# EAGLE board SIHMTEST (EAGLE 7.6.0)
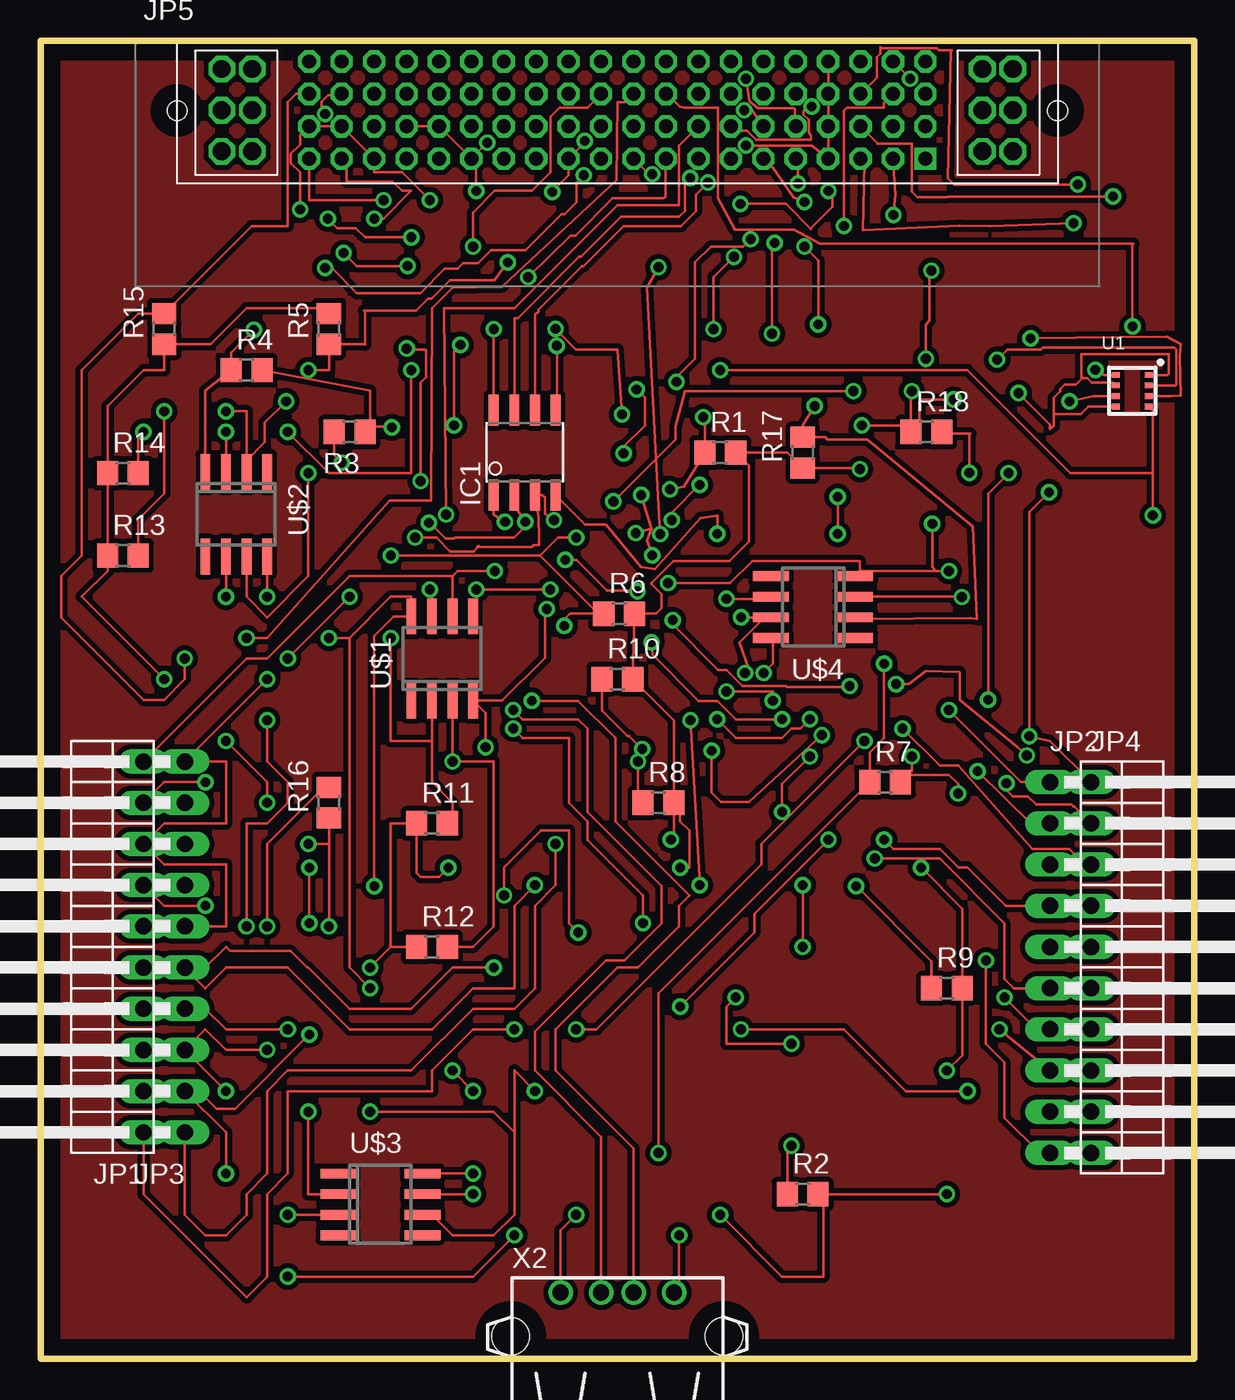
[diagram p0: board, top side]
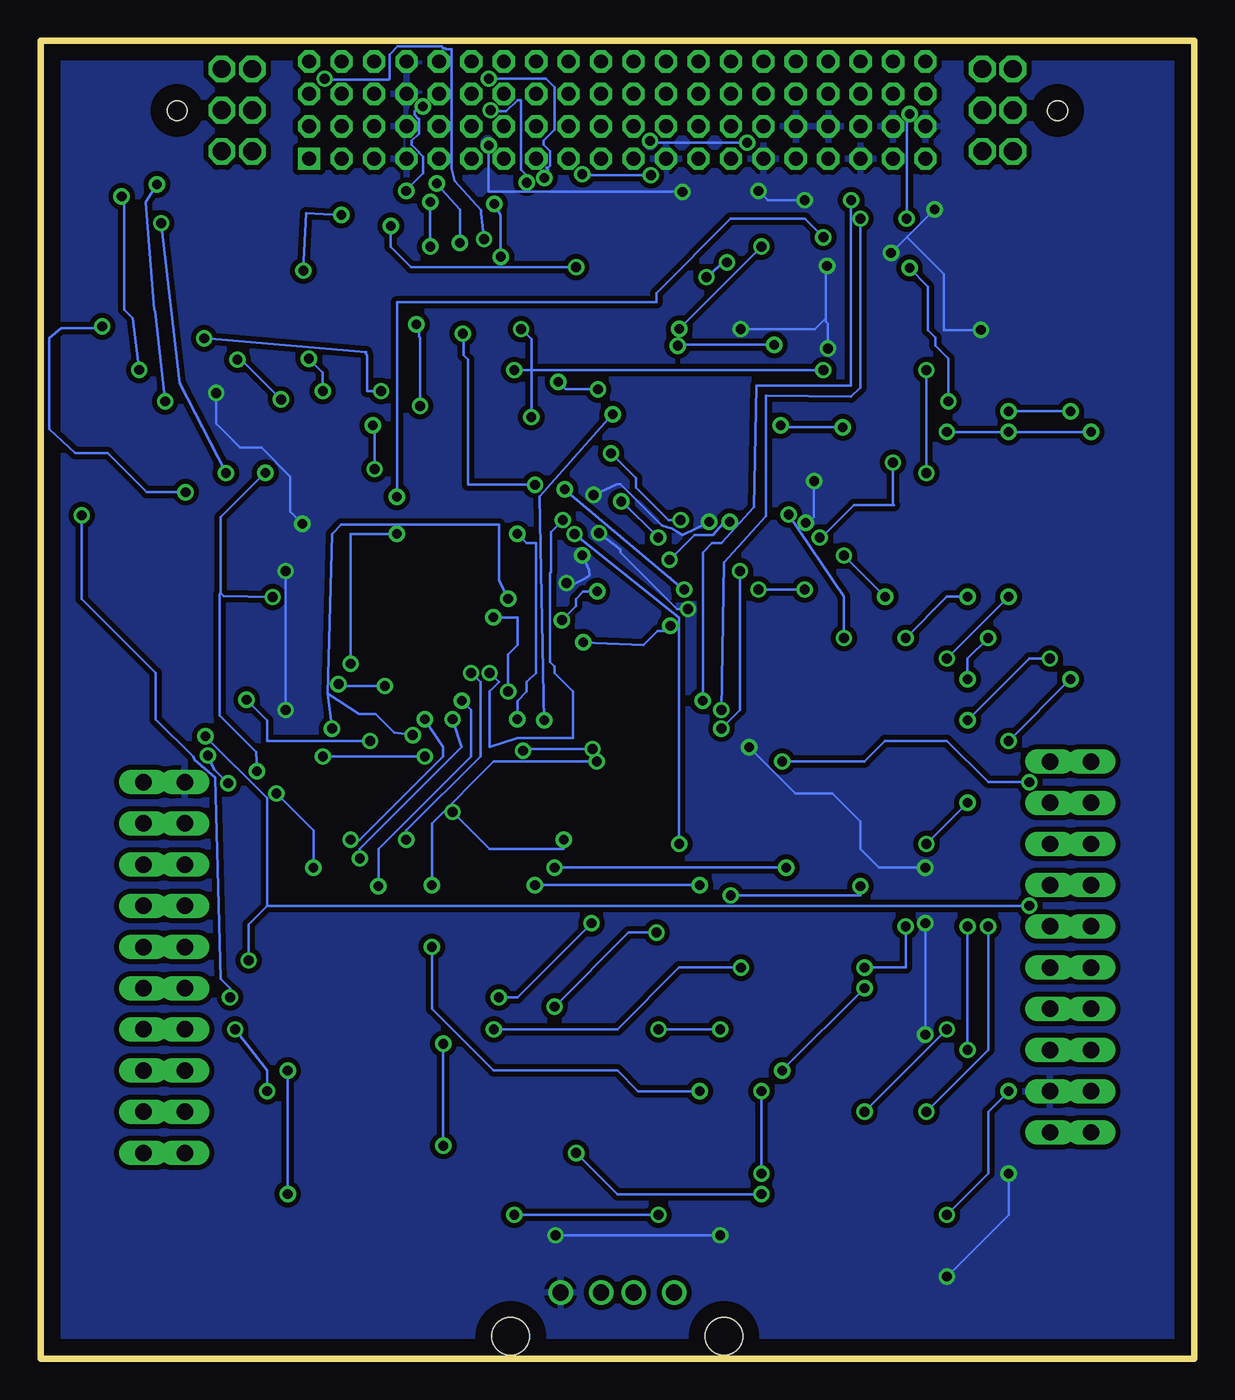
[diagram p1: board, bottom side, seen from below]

Size 71.12 x 81.28 mm. Coordinates in mm from the lower left corner, seen from the top.
Outline: 0,0 0,81.28 71.12,81.28 71.12,0 0,0
Copper layers (1*16): Top 0.035mm / dielectric 1.5mm / Bottom 0.035mm
Design rules "default": minimum track width 10mil, minimum drill 24mil, track to track 8mil, track to pad 8mil, pad to pad 8mil, via to via 8mil, smd to smd 8mil, copper to edge 40mil, drill to drill 8mil, minimum pad ring 10mil, minimum via ring 8mil, stop-mask expansion 4mil, vias tented up to drill 0mil, thermal gap 10mil

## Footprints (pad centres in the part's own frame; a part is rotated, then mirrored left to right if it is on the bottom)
SO08 = smd 0.61 x 1.905: 1 -1.905,-2.616; 2 -0.635,-2.616; 3 0.635,-2.616; 4 1.905,-2.616; 5 1.905,2.616; 6 0.635,2.616; 7 -0.635,2.616; 8 -1.905,2.616
1X10/90 = drill 1.016 long: 1 -11.43,-3.81; 2 -8.89,-3.81; 3 -6.35,-3.81; 4 -3.81,-3.81; 5 -1.27,-3.81; 6 1.27,-3.81; 7 3.81,-3.81; 8 6.35,-3.81; 9 8.89,-3.81; 10 11.43,-3.81
MPSC-01-80 = drill 0.86 square: 1 19,0.33 | drill 0.86 octagon: 2 17,0.33; 3 15,0.33; 4 13,0.33; 5 11,0.33; 6 9,0.33; 7 7,0.33; 8 5,0.33; 9 3,0.33; 10 1,0.33; 11 -1,0.33; 12 -3,0.33; 13 -5,0.33; 14 -7,0.33; 15 -9,0.33; 16 -11,0.33; 17 -13,0.33; 18 -15,0.33; 19 -17,0.33; 20 -19,0.33; 21 19,2.33; 22 17,2.33; 23 15,2.33; 24 13,2.33; 25 11,2.33; 26 9,2.33; 27 7,2.33; 28 5,2.33; 29 3,2.33; 30 1,2.33; 31 -1,2.33; 32 -3,2.33; 33 -5,2.33; 34 -7,2.33; 35 -9,2.33; 36 -11,2.33; 37 -13,2.33; 38 -15,2.33; 39 -17,2.33; 40 -19,2.33; 41 19,4.33; 42 17,4.33; 43 15,4.33; 44 13,4.33; 45 11,4.33; 46 9,4.33; 47 7,4.33; 48 5,4.33; 49 3,4.33; 50 1,4.33; 51 -1,4.33; 52 -3,4.33; 53 -5,4.33; 54 -7,4.33; 55 -9,4.33; 56 -11,4.33; 57 -13,4.33; 58 -15,4.33; 59 -17,4.33; 60 -19,4.33; 61 19,6.33; 62 17,6.33; 63 15,6.33; 64 13,6.33; 65 11,6.33; 66 9,6.33; 67 7,6.33; 68 5,6.33; 69 3,6.33; 70 1,6.33; 71 -1,6.33; 72 -3,6.33; 73 -5,6.33; 74 -7,6.33; 75 -9,6.33; 76 -11,6.33; 77 -13,6.33; 78 -15,6.33; 79 -17,6.33; 80 -19,6.33 | drill 1.1 octagon: P1,1 -24.385,0.79; P1,2 -22.505,0.79; P1,3 -24.385,3.33; P1,4 -22.505,3.33; P1,5 -24.385,5.87; P1,6 -22.505,5.87; P2,1 24.385,0.789; P2,2 22.505,0.789; P2,3 24.385,3.329; P2,4 22.505,3.329; P2,5 24.385,5.869; P2,6 22.505,5.869 | hole 1.2: -27.145,3.3; 27.145,3.3
R0805 = smd 1.3 x 1.5: 1 -0.95,0; 2 0.95,0
BME280_LGA = smd 0.5 x 0.35: P$1 1.025,0.975; P$2 1.025,0.325; P$3 1.025,-0.325; P$4 1.025,-0.975; P$5 -1.025,-0.975; P$6 -1.025,-0.325; P$7 -1.025,0.325; P$8 -1.025,0.975
SO8 = smd 0.6 x 2.2: 1 -1.905,-2.6; 2 -0.635,-2.6; 3 0.635,-2.6; 4 1.905,-2.6; 5 1.905,2.6; 6 0.635,2.6; 7 -0.635,2.6; 8 -1.905,2.6
USB = drill 1: 1 -3.5,12.99; 2 -1,12.99; 3 1,12.99; 4 3.5,12.99 | hole 2.3: -6.57,10.28; 6.57,10.28

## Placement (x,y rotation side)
IC1  MCP2551/SN  [SO08]  29.84,55.88 0 top
JP1  [1X10/90]  2.54,25.4 90 top
JP2  [1X10/90]  66.04,24.13 270 top
JP3  [1X10/90]  5.08,25.4 90 top
JP4  [1X10/90]  68.58,24.13 270 top
JP5  [MPSC-01-80]  35.56,73.66 0 top
R1  5k  [R0805]  41.91,55.88 0 top
R2  5k  [R0805]  46.99,10.16 0 top
R3  10k  [R0805]  19.05,57.15 180 top
R4  10k  [R0805]  12.7,60.96 0 top
R5  5k  [R0805]  17.78,63.5 90 top
R6  5k  [R0805]  35.67,45.95 0 top
R7  5k  [R0805]  52.07,35.56 0 top
R8  5k  [R0805]  38.1,34.29 0 top
R9  5k  [R0805]  55.88,22.86 0 top
R10  5k  [R0805]  35.56,41.91 0 top
R11  5k  [R0805]  24.13,33.02 0 top
R12  5k  [R0805]  24.13,25.4 0 top
R13  5k  [R0805]  5.08,49.53 0 top
R14  5k  [R0805]  5.08,54.61 0 top
R15  5k  [R0805]  7.62,63.5 90 top
R16  5k  [R0805]  17.78,34.29 90 top
R17  5k  [R0805]  46.99,55.88 90 top
R18  5k  [R0805]  54.61,57.15 0 top
U1  BME280  [BME280_LGA]  67.31,59.69 0 top
U$1  P82B715  [SO8]  24.77,43.18 0 top
U$2  P82B715  [SO8]  12.06,52.07 180 top
U$3  P82B715  [SO8]  20.95,9.53 270 top
U$4  P82B715  [SO8]  47.62,46.35 90 top
X2  [USB]  35.56,-8.89 0 top

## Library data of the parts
IC1 = microchip-dspic
JP1-JP4 = pinhead
JP5 = samtec
R1-R18 = resistor
U1 = BME280ComponentLibrary; PROD_ID: IC-13090
U$1-U$4 = NXP
X2 = con-amp

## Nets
3.3(1): JP1.1 JP5.3
3.3(VDDBME): JP5.23 U1.P$8
3.3(VDDIOBME): JP5.43 U1.P$6
5.0(3): JP3.1 JP5.42
5.0(BME): JP5.2 R1.2 R2.2 R5.2 R6.2 R7.2 R8.2 R9.2 R10.2 R11.1 R12.1 R13.1 R14.1 R15.1 R16.1 R17.1 R18.1 U1.P$2 X2.1
BUFFERSCL0: JP5.28 R11.2 U$1.2
BUFFERSCL1: JP5.10 R13.2 U$2.2
BUFFERSCL2: JP5.60 R15.2 U$3.2
BUFFERSCL3: JP5.6 R17.2 U$4.2
BUFFERSDA0: JP5.27 R1.1 U$1.7
BUFFERSDA1: JP5.9 R5.1 U$2.7
BUFFERSDA2: JP5.59 R7.1 U$3.7
BUFFERSDA3: JP5.5 R9.1 U$4.7
BUFFERVCC: U$1.8 U$2.8 U$3.8 U$4.8
BUFFERVCC(5V): JP5.22
CANH: IC1.7 JP5.25
CANL: IC1.6 JP5.26
CANRX: IC1.4 JP2.4
CANTX: IC1.1 JP4.2
GND: IC1.2 IC1.8 JP2.1 JP3.2 JP5.4 JP5.12 JP5.15 JP5.18 JP5.24 JP5.36 JP5.37 JP5.39 JP5.40 JP5.44 JP5.64 R4.1 U1.P$1 U1.P$5 U1.P$7 U$1.4 U$2.4 U$4.4 X2.4
GPIO_1: JP5.38
MISO: JP2.8 JP3.5 JP5.51
MOSI: JP1.8 JP3.6 JP3.10 JP5.50
N$1: JP5.1
N$2: IC1.5 R3.1 R4.2
N$7: JP5.7
N$8: JP5.8
N$11: JP5.11
N$13: JP5.13
N$14: JP5.14
N$21: JP5.21
N$29: JP5.29
N$30: JP5.30
N$31: JP5.31
N$32: JP5.32
N$33: JP5.33
N$34: JP5.34
N$35: JP5.35
N$41: JP5.41
N$45: JP5.45
N$46: JP5.46
N$47: JP5.47
N$48: JP5.48
N$52: JP5.52
N$53: JP5.53
N$54: JP5.54
N$55: JP5.55
N$56: JP5.56
N$57: JP5.57
N$58: JP5.58
N$61: JP5.61
N$63: JP5.63
N$65: JP5.65
N$66: JP5.66
N$67: JP5.67
N$68: JP5.68
N$69: JP5.69
N$70: JP5.70
N$71: JP5.71
N$72: JP5.72
N$73: JP5.73
N$74: JP5.74
N$75: JP5.75
N$76: JP5.76
N$77: JP5.77
N$78: JP5.78
N$79: JP5.79
N$80: JP5.80
PA3: JP2.9
PB5: JP1.2
PD6: JP4.8
PD7: JP4.9
PE2: JP3.8
PE3: JP3.9
PF4: JP4.10
RES: JP2.5
SPI_CLK: JP1.7 JP2.10 JP4.1 JP5.49
U1RX(USB+)-: JP1.3
U1TX(USB-)-: JP1.4
U3RX-: JP4.6
U3TX-: JP4.7
U4RX-: JP4.4
U4TX-: JP4.5
U5RX-: JP1.5
U5TX-: JP1.6
U7RX-: JP2.3
U7TX-: JP3.7
UNBUFFERSCL0: JP1.9 R12.2 U$1.3
UNBUFFERSCL1: JP2.7 R14.2 U1.P$4 U$2.3
UNBUFFERSCL2: JP3.3 R16.2 U$3.3
UNBUFFERSCL3: JP2.2 R18.2 U$4.3
UNBUFFERSDA0: JP1.10 R2.1 U$1.6
UNBUFFERSDA1: JP2.6 R6.1 U1.P$3 U$2.6
UNBUFFERSDA2: JP3.4 R8.1 U$3.6
UNBUFFERSDA3: JP4.3 R10.1 U$4.6
USB1+: JP5.17
USB1-: JP5.16
USB+: JP5.20 X2.3
USB-: JP5.19 X2.2
VDD: IC1.3 JP5.62 R3.2

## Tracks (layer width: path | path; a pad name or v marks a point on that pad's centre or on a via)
3.3(1)  (via drill 0.6)
  Top 0.152: JP1.1 6.35,10.16 12.7,3.81 13.97,5.08 13.97,10.16 15.24,11.43 15.24,16.51 24.13,16.51 24.13,17.78 26.67,20.32 v29.21,20.32 | v33.02,20.32 34.29,20.32 44.45,30.48 44.45,31.75 v50.8,38.1 | v58.42,40.64 58.42,53.34 v59.69,54.61 | v63.68,70.02 58.53,69.85 56.69,69.86 50.69,69.58 50.8,73.75 JP5.3
  Bottom 0.152: v29.21,20.32 v33.02,20.32 | v50.8,38.1 57.15,38.1 57.15,39.37 v58.42,40.64 | v59.69,54.61 62.54,60.15 v63.68,70.02
3.3(VDDBME)  (via drill 0.6)
  Top 0.152: U1.P$8 65.58,60.66 65.55,60.69 65.49,60.69 v65.04,60.98 | v66.12,71.67 55.95,71.67 55.89,71.61 54.06,71.61 53.72,71.95 53.72,74.92 51.61,74.92 51.61,74.94 JP5.23
  Bottom 0.152: v65.04,60.98 65.44,64.18 65.95,64.69 65.95,71.5 v66.12,71.67
3.3(VDDIOBME)  (via drill 0.6)
  Top 0.152: U1.P$6 64.91,59.37 v63.44,59.04 | v63.95,72.41 56.35,72.41 55.95,72.81 56.12,80.64 56.18,80.7 55.38,80.7 55.26,80.81 51.84,80.81 51.78,80.87 51.78,80.47 51.55,80.24 51.55,78.98 JP5.43
  Bottom 0.152: v63.44,59.04 64.06,64.58 64.12,64.69 64.64,71.32 v63.95,72.41
5.0(3)  (via drill 0.6)
  Top 0.152: JP3.1 8.89,8.89 10.16,7.62 11.43,7.62 12.7,8.89 12.7,10.16 13.97,11.43 13.97,16.51 15.24,17.78 22.86,17.78 26.67,21.59 29.21,21.59 30.48,22.86 30.48,27.94 31.75,29.21 v31.75,31.75 | v38.2,50.86 37.4,66.04 v38.1,67.31 | v49.53,69.85 49.53,76.96 49.72,77.15 52.01,77.15 52.01,77.44 JP5.42
  Bottom 0.152: v31.75,31.75 31.75,45.72 v38.2,50.86 | v38.1,67.31 48.26,67.31 49.53,68.58 v49.53,69.85
5.0(BME)  (via drill 0.6)
  Top 0.152: 17.36,64.77 12.7,64.77 10.48,62.55 R15.1 7.62,60.96 6.35,60.96 4.13,58.74 R14.1 R13.1 4.13,48.58 2.54,46.99 v7.62,41.91 | v11.43,38.1 13.97,35.56 v13.97,34.29 | v16.51,31.75 17.78,31.75 R16.1 v17.78,26.67 | X2.1 32.06,7.93 v33.02,8.89 | v41.91,8.89 45.72,5.08 48.26,5.08 48.26,9.84 R2.2 v55.88,10.16 | v20.32,24.13 21.59,25.4 | 21.59,25.4 R12.1 | 21.59,25.4 21.59,33.02 R11.1 23.18,29.97 23.43,29.72 24.57,29.72 v25.15,30.29 | v55.88,17.78 56.83,18.73 R9.2 56.83,27.75 v54.29,30.29 | R8.2 39.05,39.37 R10.2 R6.2 37.95,45.95 38.29,46.29 38.29,47.15 37.66,47.78 37.66,47.84 39.03,49.21 42.46,49.21 43.66,50.41 43.66,55.08 R1.2 46.04,55.88 R17.1 50.45,54.93 v50.52,54.86 | R8.2 39.43,33.91 39.43,33.15 40.01,32.58 40.01,30.29 v39.43,30.29 | R8.2 39.05,32.19 v38.86,32 | v45.72,33.72 45.72,35.43 v47.43,37.15 | v53.72,37.15 53.72,36.26 R7.2 53.47,36.01 56.01,36.01 56.58,35.43 v56.58,34.86 | U1.P$2 69.96,60.02 70.01,60.06 70.01,62.24 69.89,62.35 61.78,62.35 61.66,62.24 59.61,62.24 v58.98,61.61 | v50.63,57.55 53.26,57.55 R18.1 | v56.29,59.15 54.29,59.15 54.18,59.04 54.18,57.67 R18.1 | R18.1 53.66,59.6 v53.72,59.66 | v54.58,61.66 54.58,63.78 54.81,64.01 54.81,66.98 v54.92,67.09 | v52.58,70.52 52.71,71.78 JP5.2
  Top 0.406: 17.78,64.77 R5.2 17.36,64.77
  Bottom 0.152: v7.62,41.91 v11.43,38.1 | v13.97,34.29 v16.51,31.75 | v33.02,8.89 v41.91,8.89 | v17.78,26.67 17.78,24.13 v20.32,24.13 | v55.88,17.78 v55.88,10.16 | v25.15,30.29 v39.43,30.29 | v38.86,32 38.86,31.43 43.43,31.43 v45.72,33.72 | v54.29,30.29 54.29,32.58 v56.58,34.86 | v47.43,37.15 v53.72,37.15 | v50.52,54.86 50.52,57.44 v50.63,57.55 | v58.98,61.61 58.75,61.61 v56.29,59.15 | v53.72,59.66 53.72,60.81 v54.58,61.66 | v54.92,67.09 54.75,70.64 v52.58,70.52
5V
  pour Top (isolate 0.305): 0,81.28 0,0 71.12,0 71.12,81.28
BUFFERSCL0  (via drill 0.6)
  Top 0.152: 24.13,38.1 24.13,35.56 25.4,34.29 25.4,33.34 R11.2 | U$1.2 24.13,38.1 | 24.13,38.1 21.59,38.1 v21.59,44.45 | v25,52.06 24.89,64.77 29.21,64.77 35.56,71.12 39.37,71.12 39.37,74.8 JP5.28
  Bottom 0.152: v21.59,44.45 21.59,46.99 v25,52.06
BUFFERSCL1  (via drill 0.6)
  Top 0.152: R13.2 6.03,51.75 7.62,53.34 v7.62,58.42 | v11.43,58.42 12.7,58.42 U$2.2 12.7,55.39 13.83,56.52 13.83,57.72 v15.14,59.04 | v17.55,67.27 17.95,67.27 19.49,65.72 23.43,65.72 24.92,67.21 25.72,67.21 26.06,67.55 26.98,67.55 27.77,68.35 29.89,68.35 32.12,70.58 32.29,70.58 33.03,71.32 33.03,72.52 v33.49,72.98 | v37.72,73.04 37.51,73.04 JP5.10
  Bottom 0.152: v7.62,58.42 v11.43,58.42 | v15.14,59.04 15.14,61.66 15.95,62.47 15.95,62.98 16.4,63.44 16.4,66.12 v17.55,67.27 | v33.49,72.98 37.66,72.98 v37.72,73.04
BUFFERSCL2  (via drill 0.6)
  Top 0.152: JP5.60 15.76,77.99 15.24,77.47 15.24,69.85 13.02,69.85 R15.2 6.03,64.45 2.54,60.96 2.54,49.53 1.27,48.26 1.27,45.72 6.35,40.64 7.62,40.64 8.89,41.91 v8.89,43.18 | v13.97,39.37 13.97,36.83 15.24,35.56 15.24,34.29 13.97,33.02 12.7,33.02 v12.7,26.67 | v16.51,15.24 16.51,10.16 U$3.2
  Bottom 0.152: v8.89,43.18 10.16,43.18 v13.97,39.37 | v12.7,26.67 12.7,19.05 v16.51,15.24
BUFFERSCL3  (via drill 0.6)
  Top 0.152: v47.72,58.75 46.99,57.56 R17.2 48.38,56.83 48.52,56.69 50.98,56.69 57.49,51.32 57.72,45.61 57.32,45.66 50.34,45.61 U$4.2 | v47.95,63.78 47.95,67.72 v47.09,68.58 | v47.09,71.32 46.41,71.61 45.15,73.44 45.03,73.52 JP5.6
  Bottom 0.152: v47.72,58.75 47.72,62.98 47.78,63.04 47.78,63.61 v47.95,63.78 | v47.09,68.58 v47.09,71.32
BUFFERSDA0  (via drill 0.6)
  Top 0.152: U$1.7 24.13,47.31 v24,47.43 | v26.86,47.43 v31.43,47.43 | v38.8,53.61 39.66,53.78 R1.1 40.96,57.97 v40.86,58.06 | v41.49,63.49 41.49,66.69 v42.75,67.95 | v43.15,71.21 45.95,71.21 47.49,69.67 47.49,69.72 48.81,71.04 48.81,71.78 v48.58,72.01 | v47.55,77.21 47.32,77.15 47.03,76.92 47.03,76.69 47.38,76.41 47.38,75.61 47.49,75.44 47.49,75.15 44.12,75.15 43.55,75.72 42.83,75.72 JP5.27
  Bottom 0.152: v24,47.43 v26.86,47.43 | v31.43,47.43 31.89,47.78 v38.8,53.61 | v40.86,58.06 40.86,62.87 v41.49,63.49 | v42.75,67.95 42.75,70.52 v43.15,71.21 | v48.58,72.01 48.58,72.07 47.55,73.09 47.55,74.12 47.78,74.35 47.78,74.41 48.23,74.87 48.23,75.09 47.78,75.55 47.78,76.47 47.84,76.47 48.06,76.69 48.06,76.92 47.78,77.21 v47.55,77.21
BUFFERSDA1  (via drill 0.6)
  Top 0.152: 12.7,49.53 U$2.7 12.7,46.99 13.97,45.72 16.51,48.26 v16.51,54.61 | v16.51,60.96 17.78,60.96 R5.1 19.98,62.55 20,62.52 20,64.58 19.95,64.64 23.15,64.64 23.89,65.38 24.12,65.38 25.26,66.52 28,66.52 v28.8,67.61 | v30.06,66.69 30.12,66.75 32.69,69.27 32.98,69.27 35.26,71.55 38.41,71.55 38.52,71.67 38.52,73.95 JP5.9
  Bottom 0.152: v16.51,54.61 v16.51,60.96 | v28.8,67.61 29.09,67.55 v30.06,66.69
BUFFERSDA2  (via drill 0.6)
  Top 0.152: U$3.7 v26.67,10.16 | v38.1,12.7 38.1,22.54 R7.1 51.12,37.4 52.01,38.29 v52.01,42.86 | v49.15,50.86 v49.15,53.15 | v22.86,69.15 20,69.15 19.43,69.72 18.29,69.72 v17.72,70.29 | v17.55,76.75 17.49,76.75 17.32,76.92 17.32,77.5 17.72,77.89 18.46,77.89 JP5.59
  Bottom 0.152: v26.67,10.16 35.56,10.16 v38.1,12.7 | v52.01,42.86 52.01,50.86 v49.15,50.86 | v49.15,53.15 49.15,65.15 33.15,65.15 33.15,65.72 28.57,70.29 24,70.29 v22.86,69.15 | v17.72,70.29 17.72,76.58 v17.55,76.75
BUFFERSDA3  (via drill 0.6)
  Top 0.152: R9.1 54.93,24.51 v50.29,29.15 | v45.15,40.58 45.15,41.15 v42.29,41.15 | v43.2,45.72 44.29,45.72 44.35,45.66 44.97,45.66 U$4.7 44.63,45.72 43.09,44.18 43.66,42.52 v43.43,42.29 | v38.92,51.72 38.92,52.18 v40.63,53.89 | v45.09,63.21 45.09,68.64 v45.26,68.81 | v46.69,72.47 46.69,73.86 JP5.5
  Bottom 0.152: v50.29,29.15 50.29,31.43 44.58,37.15 44.58,40.01 v45.15,40.58 | v42.29,41.15 42.29,43.43 41.72,44.01 41.72,45.72 v43.2,45.72 | v43.43,42.29 42.86,41.72 43.43,41.15 43.43,37.72 41.72,38.29 38.29,38.29 38.29,41.15 39.43,42.29 39.43,42.69 39.72,42.98 39.72,48.46 39.66,48.52 39.66,50.98 v38.92,51.72 | v40.63,53.89 44.75,53.89 44.75,61.61 45.03,61.89 45.03,63.15 v45.09,63.21 | v45.26,68.81 45.26,70.87 v46.69,72.47
BUFFERVCC  (via drill 0.6)
  Top 0.152: U$3.8 v26.67,11.43 | 19.05,44.45 19.05,24.13 v20.32,22.86 | 19.05,44.45 21.59,46.99 22.86,46.99 U$1.8 21.78,45.78 20.57,44.58 v20.57,29.15 | U$2.8 v13.97,46.99 | v17.78,44.45 19.05,44.45 | v25.4,17.78 v26.67,16.51 | v28.57,28.57 28.57,30.29 30.86,32.58 32.58,32.58 32.58,26.86 v33.15,26.29 | v39.43,21.72 44.01,26.29 44.01,27.43 v48.58,32 | v44.58,42.29 45.15,42.86 45.15,44.33 U$4.8
  Bottom 0.152: v26.67,11.43 v26.67,16.51 | v13.97,46.99 15.24,46.99 v17.78,44.45 | v20.32,22.86 v25.4,17.78 | v20.57,29.15 20.57,28.57 v28.57,28.57 | v33.15,26.29 34.86,26.29 v39.43,21.72 | v48.58,32 48.58,32.58 44.01,37.15 44.01,41.72 v44.58,42.29
CANH  (via drill 0.6)
  Top 0.152: IC1.7 29.21,64.13 29.26,64.18 29.43,64.18 33.2,67.95 33.32,67.95 35.78,70.41 39.38,70.41 39.72,70.75 39.72,72.75 v40.06,72.81 | v43.49,78.92 43.72,77.55 44.23,77.09 46.46,77.09 46.52,77.04 46.52,76.03 JP5.25
  Bottom 0.152: v40.06,72.81 39.83,73.32 39.95,73.44 39.83,73.44 39.72,73.55 39.72,74.47 40.12,74.87 40.12,75.09 39.43,75.78 39.43,78.41 39.95,78.92 v43.49,78.92
CANL  (via drill 0.6)
  Top 0.152: IC1.6 30.48,64.37 30.69,64.58 30.69,64.69 33.38,67.38 33.49,67.38 35.95,69.84 39.49,69.84 40.41,70.75 40.41,71.78 v41.15,72.52 | v43.38,76.98 43.85,76.98 JP5.26
  Bottom 0.152: v41.15,72.52 41.15,72.98 41.49,73.32 41.49,77.61 41.72,77.61 42.41,76.92 43.03,76.92 v43.38,76.98
CANRX  (via drill 0.6)
  Top 0.152: JP2.4 59.5,27.94 57.15,30.29 56.58,30.29 55.44,31.43 52.58,31.43 v52.01,32 | v47.43,39.43 46.86,38.86 46.29,38.86 45.72,38.29 42.86,38.29 v41.72,39.43 | v41.72,50.86 41.72,52.01 40.69,51.84 37.89,48.69 37.03,48.81 34.86,51.44 33.58,51.44 IC1.4
  Bottom 0.152: v52.01,32 51.44,32 46.29,37.15 46.29,37.72 v47.43,39.43 | v41.72,39.43 41.72,40.58 41.15,41.15 41.15,41.72 40.58,42.29 40.58,50.29 41.15,50.29 v41.72,50.86
CANTX  (via drill 0.6)
  Top 0.152: IC1.1 27.94,52.07 v28.63,51.61 | v32.35,49.26 33.03,49.26 34.92,47.38 36.75,47.38 v36.8,47.32 | v38.98,45.55 38.98,45.26 41.78,42.46 42.29,42.46 43.26,41.49 45.95,41.49 46.01,41.43 49.84,41.43 v49.89,41.49 | v52.75,41.6 53.55,41.6 54.58,42.41 56.64,42.35 56.69,42.29 56.69,40.63 60.24,37.72 v60.81,37.2 | v59.55,35.49 59.55,35.09 59.95,34.69 60.87,34.69 61.38,34.18 63.55,34.18 63.66,34.06 63.73,34.06 JP4.2
  Bottom 0.152: v28.63,51.61 29.03,51.49 29.66,50.81 30.8,50.81 v32.35,49.26 | v36.8,47.32 37.66,47.32 38.12,46.86 38.12,46.41 v38.98,45.55 | v49.89,41.49 52.46,41.49 v52.75,41.6 | v60.81,37.2 60.41,36.35 v59.55,35.49
GND  (via drill 0.6)
  Top 0.152: v11.43,11.43 11.43,13.97 JP3.2 9.78,16.51 10.86,15.43 12,15.43 v16.57,20 | v15.24,5.08 26.67,5.08 v29.21,7.62 | v39.37,7.62 39.37,4.41 X2.4 | U$2.4 10.16,59.69 R4.1 11.75,62.04 v13.14,63.44 | v16.57,26.86 v16.57,30.29 | v27.43,37.72 27.43,39.82 U$1.4 28.46,40.58 31.09,43.2 31.09,46.06 31.2,46.18 v31.2,46.23 | v16,70.87 16,73.15 15.43,73.72 15.43,74.3 16,74.87 16,75.43 JP5.40 JP5.39 JP5.18 20.56,73.17 20.57,73.15 22.29,73.15 v24,71.44 | v26.86,72.01 26.86,73.69 | 26.86,73.69 JP5.15 JP5.36 JP5.37 | JP2.1 60.45,35.56 v56.01,40.01 | v56.01,48.58 55.21,48.58 | 55.21,48.58 50.54,48.58 U$4.4 50.52,48.56 50.52,49.15 50.46,49.21 43.89,49.21 42.52,47.84 v38.69,47.84 | IC1.2 29.21,52.57 v29.89,51.61 29.95,51.38 29.2,50.63 25.55,50.63 25.49,50.58 24.98,50.58 24.17,51.38 24.12,51.38 v23.95,51.55 | v23.43,54.12 23.43,60.18 23.77,60.52 23.77,62.18 23.72,62.24 22.63,62.24 v22.57,62.29 | v22.63,67.38 19.49,67.38 v18.69,68.18 | v37.03,53.26 37.66,51.21 | 37.66,51.21 37.38,50.46 v37.72,49.55 | v36.69,50.92 37.66,51.21 | JP5.64 JP5.44 JP5.24 JP5.4 47.57,74.81 v43.49,74.81 | U1.P$1 69.47,60.66 69.55,60.75 69.55,61.95 64.18,61.95 64.18,60.52 64.24,60.47 | 64.24,60.47 64.52,60.47 64.81,60.18 66.12,60.18 U1.P$7 | U1.P$5 64.6,58.72 64.12,58.24 62.47,58.24 | 62.47,58.24 62.47,59.27 62.87,59.66 62.87,59.78 63.15,60.06 63.84,60.06 64.24,60.47 | 62.47,58.24 62.47,57.55 62.24,57.32 62.24,57.61 v60.29,59.55 | v54.98,51.49 54.98,48.81 55.21,48.58 | IC1.8 v27.94,63.49 v27.95,63.49 | 26.86,73.69 26.86,74.3 v27.55,74.98 | v33.55,75.09 33.55,74.98 JP5.12 32.56,72.97 v31.55,71.95
  Bottom 0.152: v11.43,11.43 11.43,8.89 v15.24,5.08 | v29.21,7.62 v39.37,7.62 | v16.57,20 v16.57,26.86 | v16.57,30.29 19.43,30.29 20.57,31.43 20.57,33.15 22.29,34.86 24.57,34.86 v27.43,37.72 | v13.14,63.44 15.43,63.44 15.43,66.86 17.72,69.15 | 17.72,69.15 v16,70.87 | v24,71.44 26.29,71.44 v26.86,72.01 | v56.01,40.01 v56.01,48.58 | v23.95,51.55 23.77,51.55 23.43,51.89 v23.43,54.12 | v22.57,62.29 22.57,63.84 22.69,63.95 22.69,64.18 | 22.69,64.18 22.69,67.32 v22.63,67.38 | v18.69,68.18 17.72,69.15 | v31.2,46.23 31.89,46.23 35.38,49.72 35.38,49.89 v36.69,50.92 | v29.89,51.61 31.55,50.81 32.17,51.21 32.8,51.38 35.38,53.95 35.55,53.95 v37.03,53.26 | v37.72,49.55 37.32,48.63 37.26,48.29 37.55,48.12 38.23,47.78 v38.69,47.84 | v60.29,59.55 60.29,57.66 58.81,56.18 57.49,56.18 55.72,54.41 55.72,52.23 v54.98,51.49 | v27.95,63.49 23.37,63.49 22.69,64.18 | v27.55,74.98 33.43,74.98 v33.55,75.09 | v31.55,71.95 43.49,71.95 v43.49,74.81
  pour Bottom (isolate 0.305): 0,0 0,81.28 71.12,81.28 71.12,0
MISO  (via drill 0.6)
  Top 0.152: v27.94,24.13 25.4,24.13 22.86,21.59 19.05,21.59 16.51,24.13 16.45,24.13 15.43,25.15 11.68,25.15 11.43,25.4 10.16,24.13 JP3.5 10.16,22.86 11.43,24.13 15.24,24.13 19.05,20.32 24.13,20.32 26.67,22.86 29.21,22.86 29.21,27.94 v30.48,29.21 | v43.18,20.32 49.53,20.32 53.34,16.51 v57.15,16.51 | v59.12,20.32 JP2.8 | v40.64,29.21 v40.07,39.37 | v35.85,58.24 35.56,62.23 33.02,62.23 v31.75,63.5 | v26.67,68.58 26.67,70.67 28,72.01 30.29,72.01 31.43,73.15 31.43,76.58 32,77.15 33.72,77.15 JP5.51
  Bottom 0.152: v27.94,24.13 31.75,24.13 35.56,20.32 v43.18,20.32 | v57.15,16.51 57.15,17.78 v59.12,20.32 | v30.48,29.21 v40.64,29.21 | v40.07,39.37 40.35,53.16 v35.85,58.24 | v31.75,63.5 v26.67,68.58
MOSI  (via drill 0.6)
  Top 0.152: JP3.6 11.43,26.67 11.43,30.48 7.62,30.48 JP1.8 7.62,33.02 11.43,33.02 11.43,36.83 JP3.10 v13.97,41.91 | v12.7,44.45 13.97,44.45 21.53,52.93 24.07,52.93 24.13,64.77 25.4,66.04 28.47,66.1 35.5,72.68 35.56,77.47 36.04,77.47 JP5.50
  Bottom 0.152: v13.97,41.91 13.97,43.18 v12.7,44.45
N$2  (via drill 0.6)
  Top 0.152: R4.2 20.32,59.69 20.32,57.47 | 20.32,57.47 R3.1 | 20.32,57.47 21.63,57.47 v21.66,57.44 | v25.49,57.55 25.49,62.12 v25.89,62.52 | v31.83,62.47 31.83,58.58 IC1.5
  Bottom 0.152: v21.66,57.44 25.38,57.44 v25.49,57.55 | v25.89,62.52 31.77,62.52 v31.83,62.47
SPI_CLK  (via drill 0.6)
  Top 0.152: JP1.7 7.62,27.94 v10.16,27.94 | JP4.1 62.23,38.1 v60.96,38.39 60.96,52.22 v62.18,53.44 | JP2.10 61.59,12.7 59.44,14.86 59.44,18.29 58.29,19.43 v58.29,24.57 | v67.32,63.66 67.32,68.69 67.38,68.75 48.06,68.75 46.46,69.61 42.8,69.61 41.78,71.55 41.78,77.15 39.72,77.15 39.43,77.21 39.2,77.4 JP5.49
  Bottom 0.152: v10.16,27.94 57.15,27.94 | 57.15,27.94 57.15,34.58 v60.96,38.39 | v58.29,24.57 58.29,26.8 57.15,27.94 | v62.18,53.44 64.58,53.44 66.98,55.84 68.98,55.84 70.58,57.32 70.58,62.92 69.84,63.55 67.44,63.55 v67.32,63.66
UNBUFFERSCL0  (via drill 0.6)
  Top 0.152: JP1.9 7.62,35.56 v10.16,35.56 | U$1.3 v25.4,36.83 27.94,36.83 27.94,26.67 26.67,25.4 R12.2
  Bottom 0.152: v10.16,35.56 12.7,35.56 15.24,38.1 19.05,38.1 20.32,36.83 v25.4,36.83
UNBUFFERSCL1  (via drill 0.6)
  Top 0.152: R14.2 6.03,56.83 v6.35,57.15 | v11.43,57.15 U$2.3 | v22.86,60.96 22.86,54.61 17.78,54.61 v15.24,57.15 | v41.91,60.96 57.15,60.96 63.5,54.61 68.58,54.61 | 68.58,54.61 68.58,58.47 U1.P$4 | JP2.7 61.4,20.32 v59.44,22.29 | v68.58,52.01 68.58,54.61
  Bottom 0.152: v6.35,57.15 v11.43,57.15 v15.24,57.15 | v22.86,60.96 v41.91,60.96 | v59.44,22.29 59.44,22.86 60.01,23.43 60.35,35.83 61.61,36.92 61.72,37.15 64.01,39.43 64.01,42.29 68.58,46.86 v68.58,52.01
UNBUFFERSCL2  (via drill 0.6)
  Top 0.152: v11.43,16.51 JP3.3 10.16,20.32 11.43,19.05 v13.97,19.05 | v15.24,8.89 U$3.3 | R16.2 17.46,35.24 13.97,31.75 v13.97,26.67
  Bottom 0.152: v11.43,16.51 12.7,15.24 12.7,11.43 v15.24,8.89 | v13.97,26.67 v13.97,19.05
UNBUFFERSCL3  (via drill 0.6)
  Top 0.152: JP2.2 61.05,33.02 v57.78,36.23 | v57.26,54.63 57.26,56.98 57.32,57.04 55.67,57.04 R18.2 | U$4.3 56.65,46.99 v56.81,46.98
  Bottom 0.152: v57.78,36.23 57.84,37.43 60.06,39.66 60.06,47.15 60.01,47.21 | 60.01,47.21 60.01,51.89 v57.26,54.63 | v56.81,46.98 59.84,47.03 60.01,47.21
UNBUFFERSDA0  (via drill 0.6)
  Top 0.152: JP1.10 12.7,43.18 13.97,43.18 19.05,48.26 25.4,48.26 | 25.4,48.26 U$1.6 | R2.1 46.04,12.89 v46.29,13.14 | v46.29,19.43 42.29,19.43 42.29,21.72 v42.86,22.29 | v37.15,26.86 37.15,28.57 33.72,32 33.72,33.15 32.58,34.29 32.58,38.29 29.72,38.29 v29.15,38.86 | v28,48.58 25.72,48.58 25.4,48.26
  Bottom 0.152: v46.29,13.14 v46.29,19.43 | v42.86,22.29 41.72,22.29 v37.15,26.86 | v29.15,38.86 28,40.01 v28,48.58
UNBUFFERSDA1  (via drill 0.6)
  Top 0.152: U$2.6 v11.43,46.99 | v15.24,43.18 v19.05,46.99 | v21.59,49.53 30.8,49.53 | 30.8,49.53 34.38,45.95 | JP2.6 60.01,22.86 59.44,23.43 59.44,26.86 55.44,30.86 v51.44,30.86 | v37.66,44.18 37.72,43.43 40.58,40.58 41.72,40.58 42.86,39.43 v45.72,39.43 46.18,39.43 | v32.29,45.21 32.29,45.61 32.63,45.95 34.38,45.95 | 34.38,45.95 R6.1 | U1.P$3 69.71,59.37 70.29,59.38 70.24,61.84 70.29,62.58 69.44,63.04 v61.04,62.92 | v50.12,59.66 39.72,59.66 39.15,57.49 39.15,56.69 v35.32,52.86 | v33.03,50.63 31.91,50.63 30.8,49.53
  Bottom 0.152: v11.43,46.99 v15.24,43.18 | v19.05,46.99 v21.59,49.53 | v51.44,30.86 51.44,31.43 45.15,37.72 v45.72,39.43 | v37.66,44.18 33.95,44.01 33.09,44.86 32.63,44.86 v32.29,45.21 | v61.04,62.92 51.03,62.06 51.09,62.01 50.98,61.89 50.98,59.66 v50.12,59.66 | v35.32,52.86 35.26,52.86 v33.03,50.63
UNBUFFERSDA2  (via drill 0.6)
  Top 0.152: U$3.6 24.13,8.89 25.4,7.62 27.94,7.62 29.21,8.89 29.21,13.97 | 29.21,13.97 29.21,17.78 v30.48,16.51 | JP3.4 10.16,21.59 11.43,20.32 v15.24,20.32 | v20.32,15.24 27.94,15.24 29.21,13.97 | v46.99,25.4 v46.99,29.21 | v36.83,36.83 36.83,34.61 R8.1
  Bottom 0.152: v15.24,20.32 v20.32,15.24 | v30.48,16.51 34.29,16.51 35.56,17.78 43.18,17.78 46.99,21.59 v46.99,25.4 | v46.99,29.21 46.99,33.02 43.18,36.83 v36.83,36.83
UNBUFFERSDA3  (via drill 0.6)
  Top 0.152: JP4.3 64.39,30.48 63.44,31.43 61.15,31.43 56.58,36.58 55.44,36.58 v53.15,38.86 | v42.29,46.86 44.9,46.86 U$4.6 | R10.1 34.61,39.97 36.18,38.41 36.29,38.41 v37.09,37.6 | v41.38,37.49 41.38,34.92 41.95,34.35 43.66,34.35 v48.18,38.46
  Bottom 0.152: v53.15,38.86 53.44,41.03 | 53.44,41.03 53.15,50.86 52.58,51.44 42.86,51.44 42.86,48.01 v42.29,46.86 | v37.09,37.6 41.26,37.6 v41.38,37.49 | v48.18,38.46 49.32,38.63 50.46,39.78 51.49,39.78 53.44,41.03
USB+  (via drill 0.6)
  Top 0.152: X2.3 36.56,12.97 31.75,17.78 31.75,20.32 35.56,24.13 36.83,24.13 39.37,26.67 39.37,27.94 40.01,28.57 35.43,33.15 35.43,38.29 33.15,40.58 v30.29,40.58 | v21.14,71.44 16.57,71.44 16.57,73.98 JP5.20
  Bottom 0.152: v30.29,40.58 30.29,49.72 29.72,50.29 29.15,50.29 27.15,52.52 26.98,60.01 21.14,60.01 v21.14,71.44
USB-  (via drill 0.6)
  Top 0.152: X2.2 34.56,13.7 30.48,17.78 30.48,20.19 34.86,24.57 36.01,24.57 38.29,26.86 38.29,29.15 33.72,33.72 33.72,38.86 33.15,39.43 29.72,39.43 v29.15,40.01 | v20.57,70.29 21.14,70.29 22.86,72.01 22.29,72.01 21.72,72.58 18.86,72.58 18.86,73.69 JP5.19
  Bottom 0.152: v29.15,40.01 28.98,49.09 26.4,51.95 26.4,59.38 21.14,59.32 20.57,59.89 v20.57,70.29
VDD  (via drill 0.6)
  Top 0.152: R3.2 18.1,55.74 v18.57,55.26 | v23.09,50.63 24.4,50.63 25.26,49.78 26.69,49.78 27.03,50.12 26.98,50.12 26.92,50.06 30.29,50.06 30.4,50.18 30.75,50.18 30.75,50.63 30.69,51.91 IC1.3 30.92,53.26 31.09,53.09 31.09,52.12 31.38,51.84 31.55,51.84 v31.66,51.72 | v35.95,55.84 35.95,56.24 37.26,57.55 37.26,59.27 v36.75,59.78 | v39.2,60.24 39.2,60.52 40.35,61.66 40.35,67.61 41.32,68.58 43.32,68.58 v43.78,69.04 | v53.61,78.92 53.61,78.94 JP5.62
  Bottom 0.152: v18.57,55.26 18.57,52.69 18.52,52.63 20.97,52.63 22.92,50.69 23.03,50.69 v23.09,50.63 | v31.66,51.72 32.4,51.72 34.4,53.72 34.4,54.29 v35.95,55.84 | v36.75,59.78 38.75,59.78 v39.2,60.24 | v43.78,69.04 43.95,70.64 43.95,70.81 45.61,72.64 45.78,73.38 45.78,80.75 46.12,80.75 46.18,80.81 46.29,80.81 46.41,80.92 49.09,80.92 49.61,80.41 49.61,78.92 49.66,78.87 53.55,78.87 v53.61,78.92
